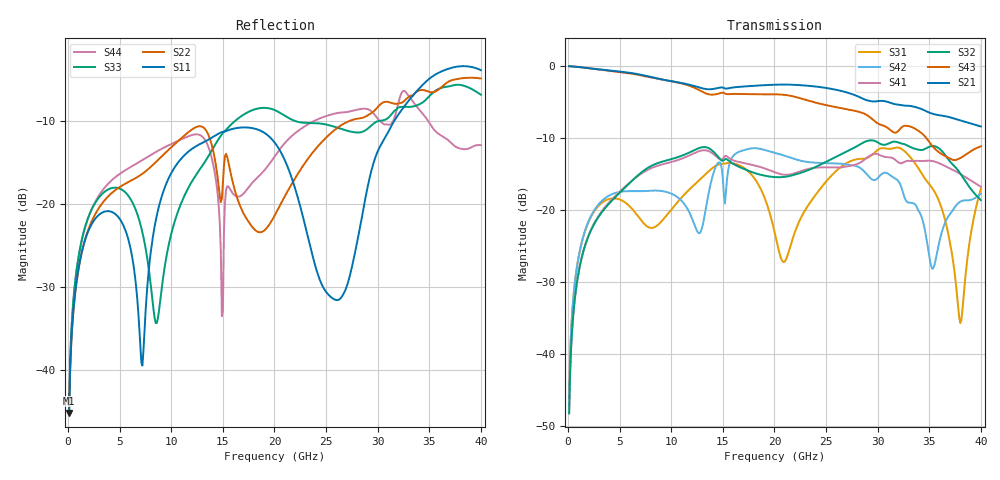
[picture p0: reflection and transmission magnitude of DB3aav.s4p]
! ADC12DJ2700AAV, ADC12DJ3200AAV, ADC08DJ3200AAV
! 144 pin AAV package
! Texas Instruments 4/21/2021
! Single-ended  S-parameters
! PORT#  PORT_NAME  NET_NAME
! PORT1:  DAxN.DIEBUMP DAxN
! PORT2:  DAxN.BGA  DAxN
! PORT3:  DAxP.DIEBUMP DAxP
! PORT4:  DAxP.BGA  DAxP
! Touchstone Ver. 1.0
! Number of ports is 4
# Hz	S	MA	R	50.000000
! SCATTERING PARAMETERS  :
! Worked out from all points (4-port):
!   400 points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, 100 MHz to 40 GHz, reference 50 ohm
!   strongest paths, dB at 100 MHz, 10.1 GHz, 20.1 GHz, 30.1 GHz, 40 GHz:
!     S21: 0.0, -2.1, -2.6, -4.9, -8.4
!     S43: 0.0, -2.1, -3.9, -8.0, -11.1
!     S32: -48.2, -12.9, -15.4, -10.7, -18.6
!     S41: -48.2, -13.3, -14.8, -12.3, -16.8
!     S42: -46.0, -17.8, -12.1, -15.4, -17.7
!     S31: -46.0, -19.8, -23.6, -11.6, -17.1
!   lowest |S11| = -45.3 dB at 100 MHz (marker M1), VSWR 1.01, Z = 50.2 + j0.502 ohm
!   |S11| at or under -10 dB: start of sweep to 31.59 GHz
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1e8  0.005458 66.3  0.9976 -1.7  0.004992 84.9  0.003888 -95.6
     0.9976 -1.7  0.005439 66.2  0.003888 -95.5  0.004989 85.6
     0.004992 84.9  0.003888 -95.5  0.006021 70.1  0.9978 -1.6
     0.003888 -95.6  0.004989 85.6  0.9978 -1.6  0.005994 70.3
2.9e9  0.08489 19.6  0.9495 -43.9  0.1061 20.4  0.08993 -154.1
       0.9495 -43.9  0.09261 26.2  0.08867 -151.5  0.1085 43.4
       0.1061 20.4  0.08867 -151.5  0.1075 20.1  0.9483 -42.7
       0.08993 -154.1  0.1085 43.4  0.9483 -42.7  0.1101 36.6
8.1e9  0.05639 66.1  0.8364 -118.4  0.07525 -162.4  0.1962 116.1
       0.8364 -118.4  0.1692 -34.3  0.2033 125.2  0.1366 1.9
       0.07525 -162.4  0.2033 125.2  0.02895 -132.1  0.832 -114.5
       0.1962 116.1  0.1366 1.9  0.832 -114.5  0.1987 -20.7
1.49e10  0.2712 -42.4  0.7108 157.5  0.2099 39.9  0.2241 -3.4
         0.7108 157.5  0.1076 -145.2  0.2205 3.0  0.1924 53.3
         0.2099 39.9  0.2205 3.0  0.2626 -0.8  0.6525 163.3
         0.2241 -3.4  0.1924 53.3  0.6525 163.3  0.02099 116.6
2.02e10  0.2262 -140.4  0.7424 87.1  0.06134 -99.6  0.1814 -80.0
         0.7424 87.1  0.08934 61.9  0.1692 -55.8  0.2478 5.5
         0.06134 -99.6  0.1692 -55.8  0.3641 -89.7  0.6358 97.2
         0.1814 -80.0  0.2478 5.5  0.6358 97.2  0.2004 23.7
2.62e10  0.02634 46.2  0.6785 -2.5  0.1933 69.4  0.1976 -155.0
         0.6785 -2.5  0.2908 -20.8  0.239 -121.0  0.2107 -16.8
         0.1933 69.4  0.239 -121.0  0.2871 -161.1  0.515 17.4
         0.1976 -155.0  0.2107 -16.8  0.515 17.4  0.3544 -37.2
4e10  0.6416 -96.4  0.3804 167.0  0.1403 113.5  0.1452 -33.9
      0.3804 167.0  0.5715 -109.4  0.1173 2.0  0.1299 19.8
      0.1403 113.5  0.1173 2.0  0.4561 -79.3  0.2773 -123.4
      0.1452 -33.9  0.1299 19.8  0.2773 -123.4  0.226 -84.3
